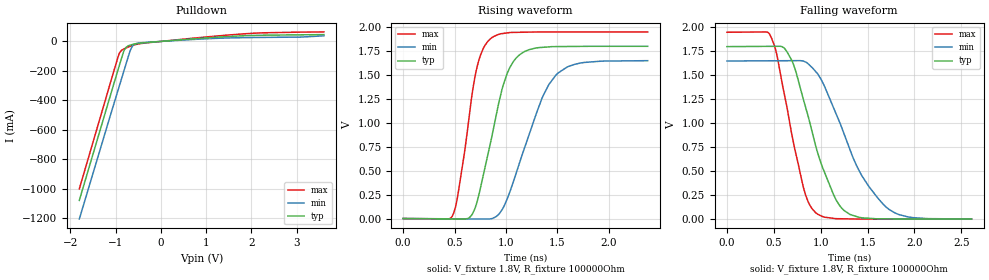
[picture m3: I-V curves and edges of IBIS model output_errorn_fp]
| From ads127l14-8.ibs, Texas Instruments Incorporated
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|   output_errorn_fp Model
[Model]   output_errorn_fp
Model_type   Open_drain
Polarity   Non-Inverting
Vmeas = 0.9
Vref = 1.8
Cref = 2pF
Rref = 100000
|   typ   min   max
C_comp   0.469pF   0.517pF   0.451pF
[Voltage Range]   1.8   1.65   1.95
[Temperature Range]   27   125   -40
[Pullup Reference]   1.8   1.65   1.95
[Pulldown Reference]   0   0   0
[Power Clamp Reference]   1.8   1.65   1.95
[GND Clamp Reference]   0   0   0
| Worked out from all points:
|   slope of the pulldown table from 0 to 0.27 V, typ, clamps not added: 39.9 ohm
|   falling waveform, V_fixture 1.8V, R_fixture 100000Ohm: 20-80 % time 331ps typ, 452ps min, 239ps max; typ from 1.8 V to 0.001 V
|   rising waveform, V_fixture 1.8V, R_fixture 100000Ohm: 20-80 % time 227ps typ, 324ps min, 161ps max; typ from 0.001 V to 1.8 V
[Pulldown]
|   Voltage   I(typ)   I(min)   I(max)
-1.8V     -1.08A     -1.206A    -1.002A
-919.8mV  -167.2mA   -305.8mA   -83.65mA
-876.6mV  -123.2mA   -262.2mA   -62.72mA
-822.6mV  -70.3mA    -207.7mA   -52.05mA
-774mV    -42.22mA   -158.8mA   -45.39mA
-671.4mV  -24.63mA   -59.11mA   -32.5mA
-639mV    -21.86mA   -38.2mA    -28.84mA
-590.4mV  -18.34mA   -21.05mA   -23.95mA
-444.6mV  -11.52mA   -9.376mA   -14.46mA
235.8mV   5.912mA    4.667mA    7.397mA
1.834V    38.58mA    25.73mA    51.48mA
3.6V      46.25mA    38.17mA    64.45mA
[Ramp]
R_load = 100000
|   typ   min   max
dV/dt_r   1.07916/2.25559e-10   0.989097/3.22334e-10   1.16921/1.6029e-10
dV/dt_f   1.07916/3.29896e-10   0.989097/4.51285e-10   1.16921/2.38544e-10
[Falling Waveform]
V_fixture = 1.8V
V_fixture_min = 1.65V
V_fixture_max = 1.95V
R_fixture = 100000Ohm
C_fixture = 0F
|   Time   V(typ)   V(min)   V(max)
0s        1.8V       1.65V      1.95V
457.8ps   1.803V     1.652V     1.926V
532.9ps   1.804V     1.653V     1.711V
696.8ps   1.645V     1.653V     860mV
839.9ps   1.164V     1.639V     248.9mV
947.7ps   760.6mV    1.538V     66.13mV
1.223ns   115.5mV    956.5mV    4.128mV
1.418ns   17.76mV    489.6mV    1.334mV
1.67ns    3.257mV    152.2mV    1.334mV
2.608ns   1.381mV    1.5mV      1.334mV
[Rising Waveform]
V_fixture = 1.8V
V_fixture_min = 1.65V
V_fixture_max = 1.95V
R_fixture = 100000Ohm
C_fixture = 0F
|   Time   V(typ)   V(min)   V(max)
0s        1.404mV    1.504mV    1.324mV
478.4ps   -2.148mV   -1.464mV   27.41mV
536.5ps   -2.579mV   -1.825mV   274.7mV
675.4ps   52.68mV    -2.687mV   1.334V
752.8ps   325.6mV    -3.167mV   1.709V
851.5ps   801.6mV    -1.052mV   1.881V
1.069ns   1.636V     377.5mV    1.945V
1.347ns   1.788V     1.249V     1.95V
1.497ns   1.797V     1.511V     1.95V
2.378ns   1.8V       1.65V      1.95V
